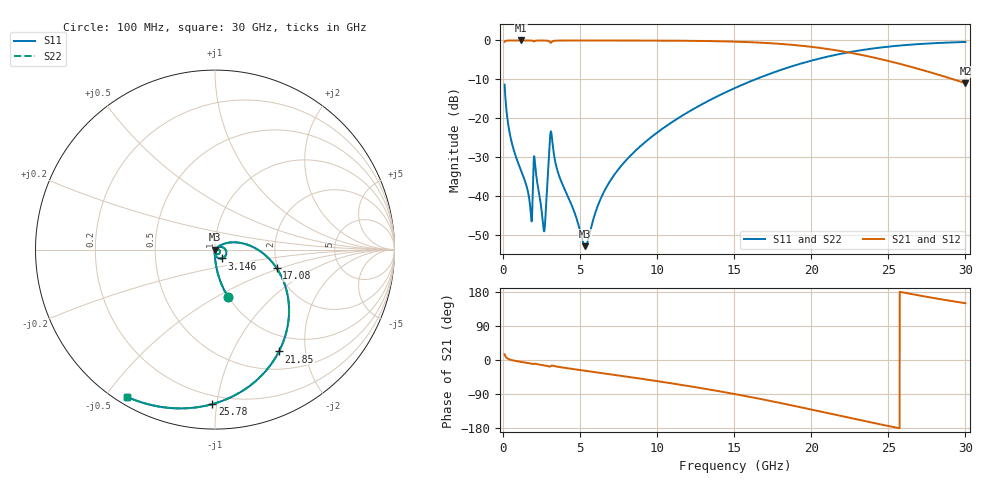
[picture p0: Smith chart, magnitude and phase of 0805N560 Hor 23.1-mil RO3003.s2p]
# GHz S MA R 50
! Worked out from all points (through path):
!   3201 points, 100 MHz to 30 GHz, reference 50 ohm
!   highest |S21| = -0.01 dB at 1.147 GHz (marker M1); lowest = -11.0 dB at 30 GHz (marker M2)
!   group delay of S21, straight-line fit = 20.3 ps
!   lowest |S11| = -52.8 dB at 5.332 GHz (marker M3), VSWR 1.00, Z = 50.2 - j0.112 ohm
!   |S11| at or under -10 dB: start of sweep to 16.36 GHz
!   |S22| runs from -52.8 to -0.4 dB; largest |S21 - S12| = 0
!   S11 on the Smith chart (normalised r, x): 100 MHz: 1.00, -0.56; 3.146 GHz: 1.07, -0.11; 17.08 GHz: 1.97, -0.47; 21.85 GHz: 0.75, -1.54; 25.78 GHz: 0.15, -0.97; 30 GHz: 0.03, -0.57
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0.1  0.2711 -74.8  0.9623 15.2  0.9623 15.2  0.2711 -74.8
0.4924375  0.0563 -88.8  0.9978 0.6  0.9978 0.6  0.0563 -88.8
1.1465  0.02198 -92.6  0.9988 -4.9  0.9988 -4.9  0.02198 -92.6
1.772531  0.006994 -80.1  0.9976 -9.1  0.9976 -9.1  0.006994 -80.1
2.108906  0.02215 -78.4  0.9915 -10.1  0.9915 -10.1  0.02215 -78.4
2.6415  0.00367 -40.6  0.9966 -14.1  0.9966 -14.1  0.00367 -40.6
2.772312  0.006531 24.5  0.9949 -15.1  0.9949 -15.1  0.006531 24.5
3.01525  0.04418 17.1  0.9632 -17.6  0.9632 -17.6  0.04418 17.1
3.146063  0.06248 -52.3  0.9497 -14.7  0.9497 -14.7  0.06248 -52.3
3.594562  0.01943 -95.5  0.9954 -18.1  0.9954 -18.1  0.01943 -95.5
5.089563  0.003063 -68.4  0.9975 -27.0  0.9975 -27.0  0.003063 -68.4
5.3325  0.002301 -28.9  0.9975 -28.4  0.9975 -28.4  0.002301 -28.9
6.210813  0.008172 39.6  0.9974 -33.4  0.9974 -33.4  0.008172 39.6
6.995687  0.01631 43.3  0.9971 -37.9  0.9971 -37.9  0.01631 43.3
10.06978  0.06744 31.1  0.9942 -56.2  0.9942 -56.2  0.06744 31.1
15.05  0.2455 -1.1  0.964 -90.0  0.964 -90.0  0.2455 -1.1
17.07759  0.3587 -16.7  0.9271 -105.8  0.9271 -105.8  0.3587 -16.7
20.03956  0.5526 -41.8  0.8257 -131.1  0.8257 -131.1  0.5526 -41.8
21.85225  0.6699 -57.8  0.7339 -147.2  0.7339 -147.2  0.6699 -57.8
25.01978  0.8325 -84.9  0.5442 -174.3  0.5442 -174.3  0.8325 -84.9
25.77662  0.8608 -90.9  0.4988 179.6  0.4988 179.6  0.8608 -90.9
30  0.9554 -120.7  0.2831 149.8  0.2831 149.8  0.9554 -120.7
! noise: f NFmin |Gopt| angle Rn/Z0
0.1  0.0003848  0.845  0.7677  0.0005273
3.417  0.01157  0.8267  18.31  0.01368
6.743  0.009807  0.6434  35.56  0.004741
10.06  0.01353  0.6275  51.83  0.005574
13.39  0.01783  0.633  67.06  0.006487
16.7  0.02305  0.6521  81.23  0.007496
20.03  0.02982  0.682  94.62  0.008698
23.35  0.0391  0.7213  107.4  0.01021
26.67  0.05275  0.7688  120.1  0.01218
30  0.07432  0.8213  132.9  0.01465
